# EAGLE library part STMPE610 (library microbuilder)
STMPE610 - 12-Bit Touch Screen Controller
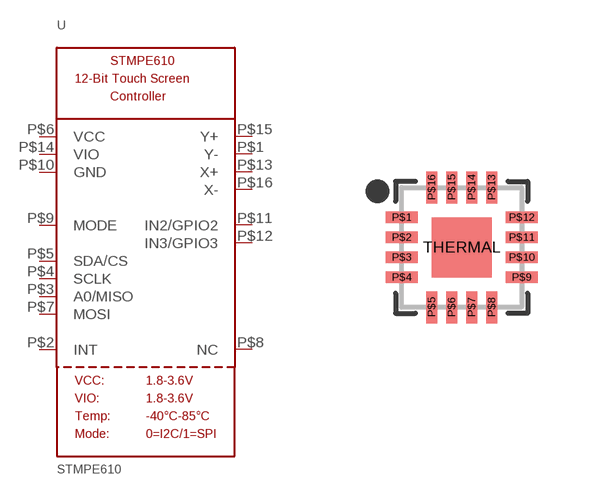
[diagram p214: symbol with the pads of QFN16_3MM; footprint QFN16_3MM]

Designator prefix U

## STMPE610  [QFN16_3MM]
P$1  Y-  in
P$2  INT  out
P$3  A0/MISO
P$4  SCLK
P$5  SDA/CS
P$6  VCC  pwr
P$7  MOSI  in
P$8  NC  nc
P$9  MODE  in
P$10  GND  pwr
P$11  IN2/GPIO2
P$12  IN3/GPIO3
P$13  X+  in
P$14  VIO  pwr
P$15  Y+  in
P$16  X-  in

## Footprint QFN16_3MM (pad centres in mm)
smd 0.8 x 0.28: P$1 -1.5,0.75; P$2 -1.5,0.25; P$3 -1.5,-0.25; P$4 -1.5,-0.75; P$9 1.5,-0.75; P$10 1.5,-0.25; P$11 1.5,0.25; P$12 1.5,0.75
smd 0.28 x 0.8: P$5 -0.75,-1.5; P$6 -0.25,-1.5; P$7 0.25,-1.5; P$8 0.75,-1.5; P$13 0.75,1.5; P$14 0.25,1.5; P$15 -0.25,1.5; P$16 -0.75,1.5
smd 1.5 x 1.5: THERMAL 0,0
